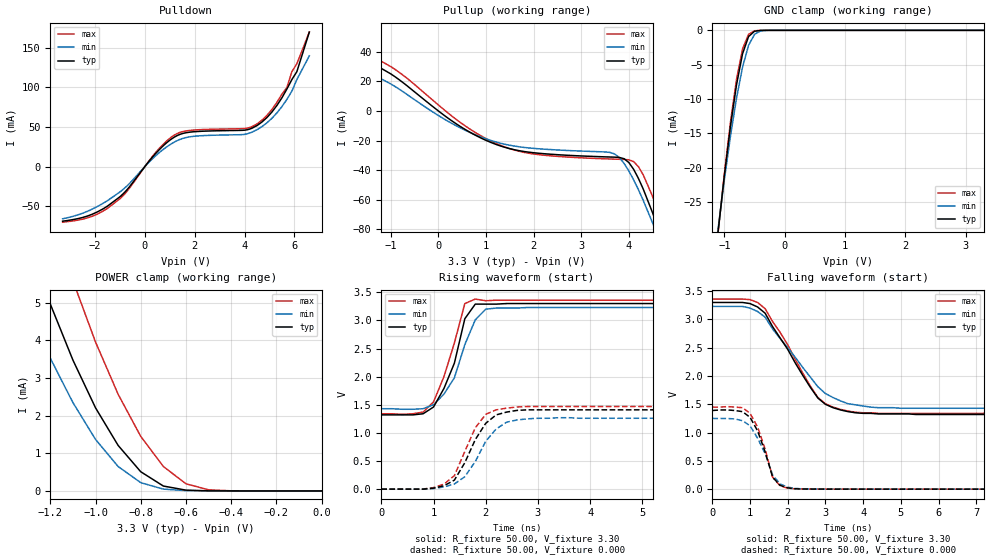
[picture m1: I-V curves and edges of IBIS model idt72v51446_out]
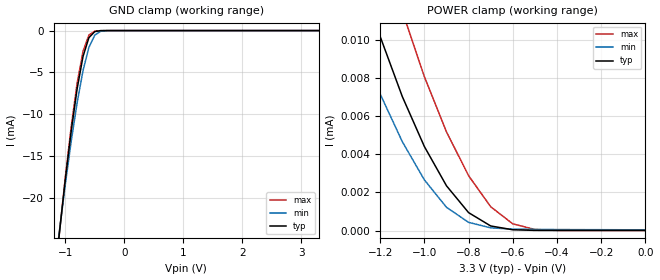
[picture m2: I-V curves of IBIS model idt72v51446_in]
| IBIS file multiq.ibs created by s2ibis2 version 1.1
| North Carolina State University Electronics Research Laboratory  1995
[IBIS ver]   3.2
[File name]   72v51446.ibs
[File Rev]   1.0
[Date]   02/11/01
[Source]   Integrated Device Technology, Inc.
[Notes]   1.Temperatures: typ=25C, min=100C, max=0C 2.Cemos11.5_sac
   3.3vv process. 3.RRmp rates based on 50 ohm load.
[Disclaimer] Integrated Device Technology, Inc. ("IDT") hereby grants the
   user of this IBIS model a non-exclusive, nontransferable
   license to use this IBIS model under the following terms. The
   user is granted this license only to use the IBIS model and is
   not granted rights to sell, copy (except as needed to run the
   IBIS model), rent, lease or sub-license the IBIS model in
   whole or in part, or in modified form to anyone. The User may
   modify the IBIS model to suit its specific applications, but
   rights to derivative works and such modifications shall belong
   to IDT. This IBIS model is provided on an AS IS" basis and IDT
   makes absolutely no warranty with respect to the information
   contained herein. IDT DISCLAIMS AND CUSTOMER WAIVES ALL
   WARRANTIES, EXPRESS AND IMPLIED, INCLUDING WARRANTIES OF
   MERCHANTABILITY AND FITNESS FOR A PARTICULAR PURPOSE. THE
   ENTIRE RISK AS TO QUALITY AND PERFORMANCE IS WITH THE USER
   ACCORDINGLY, IN NO EVENT SHALL IDT BE LIABLE FOR ANY DIRECT OR
   INDIRECT DAMAGES, WHETHER IN CONTRACT OR TORT, INCLUDING A
[Copyright]   Copyright 1999, Integrated Device Technology, Inc. all rights
   reserved
|   Component multiq
[Component]   multiq
[Manufacturer]   Integrated Device Technology
[Package]
| variable   typ   min   max
R_pkg   0.15   0.13   0.19
L_pkg   4.00nH   3.65nH   6.07nH
C_pkg   1.40pF   1.28pF   1.66pF
[Pin]  signal_name   model_name   R_pin   L_pin   C_pin
A1   D14   idt72v51446_in
A2   D13   idt72v51446_in
A3   D12   idt72v51446_in
A4   D10   idt72v51446_in
A5   D7   idt72v51446_in
A6   D4   idt72v51446_in
A7   D1   idt72v51446_in
A8   TCK   idt72v51446_in
A9   TDO   idt72v51446_out
A10   ID1   idt72v51446_in
A11   Q3   idt72v51446_out
A12   Q6   idt72v51446_out
A13   Q9   idt72v51446_out
A14   Q12   idt72v51446_out
A15   Q14   idt72v51446_out
A16   Q15   idt72v51446_out
B1   D15   idt72v51446_in
B2   D16   idt72v51446_in
B3   D11   idt72v51446_in
B4   D9   idt72v51446_in
B5   D6   idt72v51446_in
B6   D3   idt72v51446_in
B7   D0   idt72v51446_in
B8   TMS   idt72v51446_in
B9   TDI   idt72v51446_in
B10   ID0   idt72v51446_in
B11   Q2   idt72v51446_out
B12   Q5   idt72v51446_out
B13   Q8   idt72v51446_out
B14   Q11   idt72v51446_out
B15   Q13   idt72v51446_out
B16   Q19   idt72v51446_out
C1   D17   idt72v51446_in
C2   D18   idt72v51446_in
C3   D19   idt72v51446_in
C4   D8   idt72v51446_in
C5   D5   idt72v51446_in
C6   D2   idt72v51446_in
C7   TRST   idt72v51446_in
C8   IQSEL   idt72v51446_in
C9   ID2   idt72v51446_in
C10   Q0   idt72v51446_out
C11   Q1   idt72v51446_out
C12   Q4   idt72v51446_out
C13   Q7   idt72v51446_out
C14   Q10   idt72v51446_out
C15   Q17   idt72v51446_out
C16   Q18   idt72v51446_out
D1   D20   idt72v51446_in
D2   D21   idt72v51446_in
D3   D22   idt72v51446_in
D4   VDD   POWER
D5   VDD   POWER
D6   VDD   POWER
D7   VDD   POWER
D8   VDD   POWER
D9   VDD   POWER
D10   VDD   POWER
D11   VDD   POWER
D12   VDD   POWER
D13   VDD   POWER
D14   Q16   idt72v51446_out
D15   Q21   idt72v51446_out
D16   Q20   idt72v51446_out
E1   D23   idt72v51446_in
E2   D24   idt72v51446_in
E3   D24   idt72v51446_in
E4   VDD   POWER
E5   VDD   POWER
E6   VDD   POWER
E7   VDD   POWER
E8   GND   GND
E9   GND   GND
E10   VDD   POWER
E11   VDD   POWER
E12   VDD   POWER
E13   VDD   POWER
E14   Q24   idt72v51446_out
E15   Q23   idt72v51446_out
E16   Q22   idt72v51446_out
F1   D26   idt72v51446_in
F2   D27   idt72v51446_in
F3   D28   idt72v51446_in
F4   VDD   POWER
F5   VDD   POWER
F6   GND   GND
F7   GND   GND
F8   GND   GND
F9   GND   GND
F10   GND   GND
F11   GND   GND
F12   VDD   POWER
F13   VDD   POWER
F14   Q27   idt72v51446_out
F15   Q26   idt72v51446_out
F16   Q25   idt72v51446_out
G1   D29   idt72v51446_in
G2   D30   idt72v51446_in
G3   D31   idt72v51446_in
G4   VDD   POWER
G5   VDD   POWER
G6   GND   GND
G7   GND   GND
G8   GND   GND
G9   GND   GND
G10   GND   GND
G11   GND   GND
G12   VDD   POWER
G13   VDD   POWER
G14   Q30   idt72v51446_out
G15   Q29   idt72v51446_out
G16   Q28   idt72v51446_out
H1   D32   idt72v51446_in
H2   D33   idt72v51446_in
H3   D34   idt72v51446_in
H4   VDD   POWER
H5   GND   GND
H6   GND   GND
H7   GND   GND
H8   GND   GND
H9   GND   GND
H10   GND   GND
H11   GND   GND
H12   GND   GND
H13   VDD   POWER
H14   Q33   idt72v51446_out
H15   Q32   idt72v51446_out
H16   Q31   idt72v51446_out
J1   GND   GND
J2   GND   GND
J3   D35   idt72v51446_in
J4   VDD   POWER
J5   GND   GND
J6   GND   GND
J7   GND   GND
J8   GND   GND
J9   GND   GND
J10   GND   GND
J11   GND   GND
J12   GND   GND
J13   VDD   POWER
J14   PKT   idt72v51446_in
J15   Q35   idt72v51446_out
J16   Q34   idt72v51446_out
K1   PD   idt72v51446_in
K2   GND   GND
K3   VREF   POWER
K4   VDD   POWER
K5   VDD   POWER
K6   GND   GND
K7   GND   GND
K8   GND   GND
K9   GND   GND
K10   GND   GND
K11   GND   GND
K12   VDD   POWER
K13   VDD   POWER
K14   GND   GND
K15   MASTER   idt72v51446_in
K16   FM   idt72v51446_in
L1   SI   idt72v51446_in
L2   DFM   idt72v51446_in
L3   DF   idt72v51446_in
L4   VDD   POWER
L5   VDD   POWER
L6   GND   GND
L7   GND   GND
L8   GND   GND
L9   GND   GND
L10   GND   GND
L11   GND   GND
L12   VDD   POWER
L13   VDD   POWER
L14   BM   idt72v51446_in
L15   IW   idt72v51446_in
L16   OW   idt72v51446_in
M1   SENBO   idt72v51446_out
M2   SENBI   idt72v51446_in
M3   SO   idt72v51446_out
M4   VDD   POWER
M5   VDD   POWER
M6   VDD   POWER
M7   VDD   POWER
M8   GND   GND
M9   GND   GND
M10   VDD   POWER
M11   VDD   POWER
M12   VDD   POWER
M13   VDD   POWER
M14   OEX   idt72v51446_in
M15   RDADD0   idt72v51446_in
M16   RDADD1   idt72v51446_in
N1   WRADD1   idt72v51446_in
N2   WRADD0   idt72v51446_in
N3   SCLK   idt72v51446_in
N4   VDD   POWER
N5   VDD   POWER
N6   VDD   POWER
N7   VDD   POWER
N8   VDD   POWER
N9   VDD   POWER
N10   VDD   POWER
N11   VDD   POWER
N12   VDD   POWER
N13   VDD   POWER
N14   RDADD2   idt72v51446_in
N15   RDADD3   idt72v51446_in
N16   RDADD4   idt72v51446_in
P1   WRADD4   idt72v51446_in
P2   WRADD3   idt72v51446_in
P3   WRADD2   idt72v51446_in
P4   WADEN   idt72v51446_in
P5   PAF3   idt72v51446_out
P6   PAF6   idt72v51446_out
P7   PAF7   idt72v51446_out
P8   FFX   idt72v51446_out
P9   OVX   idt72v51446_out
P10   AEX   idt72v51446_out
P11   PAE7   idt72v51446_out
P12   PAE6   idt72v51446_out
P13   PAE3   idt72v51446_out
P14   RDADD5   idt72v51446_in
P15   RDADD6   idt72v51446_in
P16   RDADD7   idt72v51446_in
R1   WRADD6   idt72v51446_in
R2   WRADD5   idt72v51446_in
R3   FSYNC   idt72v51446_out
R4   FSTR   idt72v51446_in
R5   PAF2   idt72v51446_out
R6   PAF5   idt72v51446_out
R7   PAF4   idt72v51446_out
R8   AFX   idt72v51446_out
R9   PRX   idt72v51446_out
R10   ERCLK   idt72v51446_out
R11   ERENB   idt72v51446_out
R12   PAE5   idt72v51446_out
R13   PAE2   idt72v51446_out
R14   RADEN   idt72v51446_in
R15   ESTR   idt72v51446_in
R16   ESYNC   idt72v51446_out
T1   WRADD7   idt72v51446_in
T2   FXI   idt72v51446_in
T3   FXO   idt72v51446_out
T4   PAF0   idt72v51446_out
T5   PAF1   idt72v51446_out
T6   WENX   idt72v51446_in
T7   WCLK   idt72v51446_in
T8   PRSX   idt72v51446_in
T9   MRSX   idt72v51446_in
T10   RCLK   idt72v51446_in
T11   RENX   idt72v51446_in
T12   PAE4   idt72v51446_out
T13   PAE1   idt72v51446_out
T14   PAE0   idt72v51446_out
T15   EXO   idt72v51446_out
T16   EXI   idt72v51446_in
| Models and submodels in the file (2): idt72v51446_out (3-state), idt72v51446_in (Input)
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| in   in   dummy_model
| oe   oe   dummy_model
|   Model idt72v51446_out
[Model]   idt72v51446_out
Model_type   3-state
Polarity   Non-Inverting
Enable   Active-High
Vmeas =   1.50V
C_comp   3.00pF   NA   NA
[Temperature Range]   25.00   100.00   0.000
[Voltage Range]   3.30V   3.15V   3.45V
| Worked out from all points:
|   slope of the pulldown table from 0 to 0.495 V, typ, clamps not added: 26.6 ohm
|   slope of the pullup table from 0 to 0.495 V, typ, clamps not added: 44.2 ohm
|   GND clamp passes 1 mA (typ) near -0.60 V on its own axis
|   POWER clamp passes 1 mA (typ) near -0.87 V on its own axis
|   rising waveform, R_fixture 50.00, V_fixture 3.30: 20-80 % time 413ps typ, 467ps min, 415ps max; typ from 1.32 V to 3.3 V
|   rising waveform, R_fixture 50.00, V_fixture 0.000: 20-80 % time 492ps typ, 520ps min, 447ps max; typ from 0 V to 1.41 V
|   falling waveform, R_fixture 50.00, V_fixture 3.30: 20-80 % time 1.12ns typ, 1.27ns min, 1.07ns max; typ from 3.3 V to 1.32 V
|   falling waveform, R_fixture 50.00, V_fixture 0.000: 20-80 % time 438ps typ, 491ps min, 418ps max; typ from 1.39 V to 0 V
[Pulldown]
| voltage   I(typ)   I(min)   I(max)
-3.3V     -69mA      -66mA      -70.3mA
-2.1V     -60.1mA    -53.6mA    -62.7mA
-1V       -38.17mA   -32.09mA   -40.67mA
500mV     18.81mA    15.51mA    20.2mA
1.3V      39.25mA    32.83mA    41.78mA
4.1V      46.49mA    41.39mA    48.49mA
4.7V      56.32mA    50.52mA    58.66mA
5.3V      77.29mA    67.89mA    81.16mA
5.7V      98.06mA    84.95mA    100mA
5.9V      110mA      95.35mA    120mA
6.1V      120mA      110mA      130mA
6.6V      170mA      140mA      170mA
[Pullup]
| voltage   I(typ)   I(min)   I(max)
-3.3V     53.57mA    46.6mA     56.76mA
-1.5V     34.42mA    26.79mA    39.1mA
-800mV    20.6mA     14.28mA    25.63mA
300mV     -7.09mA    -8.74mA    -3.9mA
1.2V      -22.53mA   -20.92mA   -21.84mA
2V        -28.28mA   -25.32mA   -29.13mA
3.7V      -31.27mA   -29.08mA   -32.6mA
4V        -34.94mA   -40.7mA    -33.07mA
4.2V      -45.65mA   -53.32mA   -37.71mA
4.5V      -69.18mA   -76mA      -58.07mA
4.7V      -87.32mA   -92.7mA    -75.85mA
6.6V      -280mA     -270mA     -270mA
[GND_clamp]
| voltage   I(typ)   I(min)   I(max)
-3.3V     -250mA     -230mA     -250mA
-1.1V     -28.93mA   -28.53mA   -29.06mA
-1V       -21.08mA   -21.69mA   -20.81mA
-900mV    -13.99mA   -15.43mA   -13.39mA
-800mV    -7.96mA    -9.91mA    -7.17mA
-700mV    -3.43mA    -5.38mA    -2.73mA
-600mV    -910uA     -2.19mA    -580uA
-500mV    -130uA     -570uA     -63.52uA
-400mV    -11.23uA   -91.79uA   -4.22uA
-300mV    -650nA     -10.84uA   -170nA
3.3V      430pA      38.95nA    67.3pA
[POWER_clamp]
| voltage   I(typ)   I(min)   I(max)
-3.3V     67.53mA    55.8mA     76.44mA
-1.4V     8.58mA     6.43mA     11.76mA
-1.3V     6.68mA     4.9mA      9.51mA
-1.2V     4.97mA     3.53mA     7.45mA
-1.1V     3.48mA     2.35mA     5.59mA
-1V       2.21mA     1.37mA     3.96mA
-900mV    1.21mA     650uA      2.57mA
-800mV    510uA      220uA      1.45mA
-700mV    130uA      48.22uA    650uA
-600mV    20.84uA    7.95uA     190uA
-500mV    2.28uA     1.14uA     29.66uA
0V        430pA      34.34nA    100pA
[Ramp]
| variable   typ   min   max
dV/dt_r   0.85/0.46n   0.76/0.50n   0.88/0.42n
dV/dt_f   1.19/1.14n   1.08/1.32n   1.22/1.10n
R_load = 50.00
[Rising Waveform]
R_fixture = 50.00
V_fixture = 3.30
V_fixture_min = 3.15
V_fixture_max = 3.45
R_dut = 0.16
L_dut = 4.86nH
C_dut = 1.47pF
| time   V(typ)   V(min)   V(max)
0s        1.32V      1.43V      1.34V
800ps     1.34V      1.43V      1.37V
1ns       1.46V      1.5V       1.55V
1.2ns     1.79V      1.69V      2V
1.4ns     2.24V      1.98V      2.6V
1.6ns     3.03V      2.57V      3.3V
1.8ns     3.29V      3.01V      3.38V
2ns       3.29V      3.2V       3.35V
2.2ns     3.29V      3.22V      3.36V
10ns      3.3V       3.23V      3.36V
[Rising Waveform]
R_fixture = 50.00
V_fixture = 0.000
V_fixture_min = 0.000
V_fixture_max = 0.000
R_dut = 0.16
L_dut = 4.86nH
C_dut = 1.47pF
| time   V(typ)   V(min)   V(max)
0s        0V         1.6uV      0V
1ns       16.97mV    10.77mV    26.65mV
1.4ns     160mV      91.16mV    240mV
1.6ns     470mV      220mV      670mV
1.8ns     880mV      490mV      1.09V
2ns       1.17V      850mV      1.33V
2.2ns     1.32V      1.07V      1.41V
2.4ns     1.37V      1.19V      1.44V
3.4ns     1.41V      1.27V      1.47V
10ns      1.41V      1.26V      1.47V
[Falling Waveform]
R_fixture = 50.00
V_fixture = 3.30
V_fixture_min = 3.15
V_fixture_max = 3.45
R_dut = 0.16
L_dut = 4.86nH
C_dut = 1.47pF
| time   V(typ)   V(min)   V(max)
0s        3.3V       3.23V      3.36V
1ns       3.28V      3.2V       3.35V
1.4ns     3.11V      3.04V      3.19V
1.6ns     2.87V      2.83V      2.96V
2ns       2.47V      2.5V       2.55V
2.8ns     1.61V      1.81V      1.62V
3.2ns     1.44V      1.62V      1.45V
3.6ns     1.37V      1.51V      1.38V
4.4ns     1.33V      1.44V      1.34V
10ns      1.32V      1.43V      1.34V
[Falling Waveform]
R_fixture = 50.00
V_fixture = 0.000
V_fixture_min = 0.000
V_fixture_max = 0.000
R_dut = 0.16
L_dut = 4.86nH
C_dut = 1.47pF
| time   V(typ)   V(min)   V(max)
0s        1.39V      1.25V      1.45V
800ps     1.37V      1.21V      1.44V
1ns       1.27V      1.12V      1.34V
1.2ns     1.03V      900mV      1.1V
1.4ns     660mV      630mV      710mV
1.6ns     210mV      250mV      210mV
1.8ns     66.29mV    90.44mV    56.75mV
2ns       22.19mV    34.77mV    17.86mV
2.6ns     1.81mV     2.13mV     1.67mV
10ns      0V         730nV      0V
|   Model idt72v51446_in
[Model]   idt72v51446_in
Model_type   Input
Vinl =   0.80V
Vinh =   2.00V
Vmeas =   1.50V
C_comp   3.00pF   NA   NA
[Temperature Range]   25.00   100.00   0.000
[Voltage Range]   3.30V   3.15V   3.45V
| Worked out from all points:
|   GND clamp passes 1 mA (typ) near -0.61 V on its own axis
[GND_clamp]
| voltage   I(typ)   I(min)   I(max)
-3.3V     -190mA     -180mA     -200mA
-1.1V     -24.11mA   -23.92mA   -24.16mA
-1V       -17.78mA   -18.35mA   -17.52mA
-900mV    -11.99mA   -13.21mA   -11.47mA
-800mV    -6.97mA    -8.63mA    -6.3mA
-700mV    -3.1mA     -4.79mA    -2.48mA
-600mV    -850uA     -2.01mA    -540uA
-500mV    -120uA     -540uA     -60.75uA
-400mV    -10.83uA   -87.7uA    -4.08uA
-300mV    -630nA     -10.35uA   -170nA
3.3V      3.73nA     42.17nA    3.36nA
[POWER_clamp]
| voltage   I(typ)   I(min)   I(max)
-3.3V     160uA      140uA      190uA
-1.4V     17.9uA     13.4uA     24.81uA
-1.3V     13.82uA    10.09uA    19.92uA
-1.2V     10.19uA    7.17uA     15.48uA
-1.1V     7.04uA     4.67uA     11.52uA
-1V       4.41uA     2.66uA     8.08uA
-900mV    2.35uA     1.22uA     5.18uA
-800mV    940nA      430nA      2.88uA
-700mV    240nA      140nA      1.25uA
-600mV    39.61nA    73.27nA    350nA
-500mV    8.26nA     57.75nA    56.48nA
0V        3.73nA     37.83nA    3.52nA
